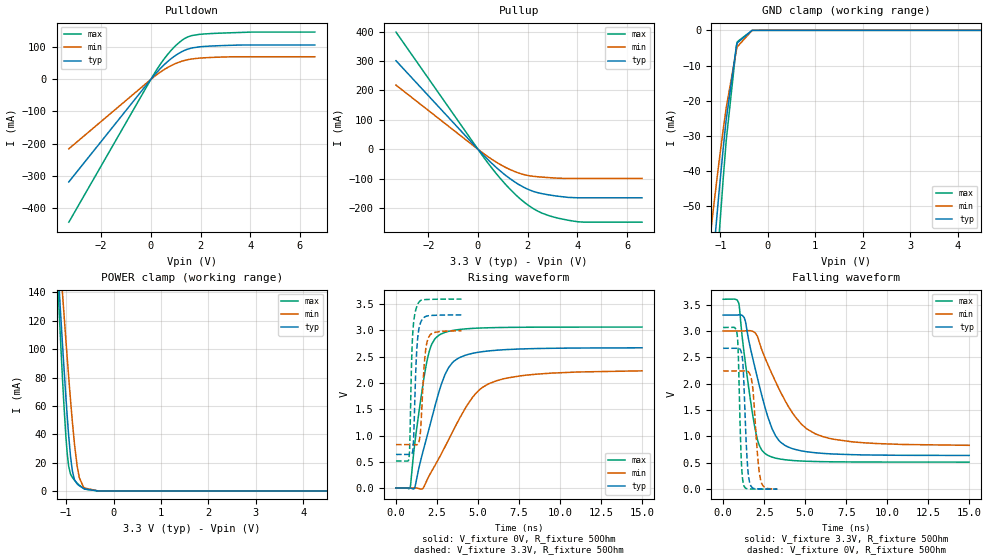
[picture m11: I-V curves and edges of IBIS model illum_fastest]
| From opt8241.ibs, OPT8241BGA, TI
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|   illum_fastest Model
[Model]   illum_fastest
Model_type   I/O
Polarity   Non-Inverting
Enable   Active-High
Vinl  = 0.99
Vinh  = 2.31
Vmeas = 1.65
Vref  = 0
Cref  = 2pF
Rref  = 50
|   typ   min   max
|   (nom PVT)   (fast PVT)   (slow PVT)
C_comp   2.708e-12   2.507e-12   2.914e-12
[Model spec]
|subparameter
Vinl   0.99   0.90   1.08
Vinh   2.31   2.10   2.52
| Where nom  PVT is Nominal Process, 3.3V, 27C
|   Fast PVT is Strong Process,  3.6V, -40C
|   Slow PVT is Weak Process,   3V, 125C
[Voltage Range]   3.3   3   3.6
|Junction Temperature
[Temperature Range]   27   125   -40
[Pullup Reference]   3.3   3   3.6
[Pulldown Reference]   0   0   0
[Power Clamp Reference]   3.3   3   3.6
[GND Clamp Reference]   0   0   0
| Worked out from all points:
|   slope of the pulldown table from 0 to 0.495 V, typ, clamps not added: 11.6 ohm
|   slope of the pullup table from 0 to 0.495 V, typ, clamps not added: 11.6 ohm
|   falling waveform, V_fixture 3.3V, R_fixture 50Ohm: 20-80 % time 1.36ns typ, 2.23ns min, 828ps max; typ from 3.3 V to 0.64 V
|   rising waveform, V_fixture 0V, R_fixture 50Ohm: 20-80 % time 1.44ns typ, 2.41ns min, 853ps max; typ from 0 V to 2.67 V
|   rising waveform, V_fixture 3.3V, R_fixture 50Ohm: 20-80 % time 199ps typ, 252ps min, 166ps max; typ from 0.639 V to 3.3 V
|   falling waveform, V_fixture 0V, R_fixture 50Ohm: 20-80 % time 221ps typ, 314ps min, 165ps max; typ from 2.67 V to 0.001 V
[Pulldown]
|   Voltage   I(typ)   I(min)   I(max)
-3.3V     -319.9mA   -216.5mA   -445.5mA
189mV     17.58mA    11.85mA    24.51mA
462mV     40.27mA    27mA       56.22mA
775.2mV   62.22mA    41.4mA     87.06mA
1.056V    78.05mA    51.51mA    109.5mA
1.251V    86.82mA    56.93mA    122mA
1.596V    97.13mA    63.25mA    135.8mA
2.165V    103mA      67.59mA    142mA
4.032V    107.5mA    70.78mA    147.8mA
6.6V      107.5mA    70.78mA    147.8mA
[GND Clamp]
|   Voltage   I(typ)   I(min)   I(max)
-3.3V     -1.553A    -1.315A    -1.789A
-1.214V   -75.2mA    -58.77mA   -96.04mA
-1.133V   -62.06mA   -49.14mA   -79.22mA
-1.033V   -46.78mA   -37.93mA   -59.46mA
-940.5mV  -33.68mA   -28.26mA   -42.33mA
-876mV    -25.29mA   -22mA      -31.29mA
-663mV    -4.673mA   -5.695mA   -4.527mA
-643.2mV  -3.575mA   -4.674mA   -3.252mA
-330mV    -4.518uA   -17.28uA   -5.664uA
6.6V      0A         0A         0A
[Pullup]
|   Voltage   I(typ)   I(min)   I(max)
-3.3V     301mA      218.2mA    398.3mA
1.2mV     -109.4uA   -79.25uA   -144.7uA
459mV     -39.81mA   -28.44mA   -53.04mA
855mV     -70.54mA   -49.65mA   -94.7mA
1.251V    -97.42mA   -67.29mA   -132mA
1.899V    -131.4mA   -86.9mA    -182.2mA
2.237V    -143.2mA   -91.82mA   -202mA
2.565V    -150.5mA   -94.39mA   -216.4mA
3.032V    -157.2mA   -97.16mA   -229.8mA
3.633V    -163.4mA   -99.07mA   -241mA
4.3V      -164.7mA   -99.07mA   -247.6mA
6.6V      -164.7mA   -99.07mA   -247.6mA
[POWER Clamp]
|   Voltage   I(typ)   I(min)   I(max)
-3.3V     1.469A     1.283A     1.789A
-1.219V   185.1mA    209mA      179.1mA
-1.136V   137.8mA    168.8mA    120.5mA
-1.068V   100mA      136.4mA    75.26mA
-1.007V   68.16mA    108.2mA    40.34mA
-973.5mV  52.09mA    93.27mA    25.99mA
-942mV    38.22mA    79.55mA    17.05mA
-867.9mV  14.43mA    49.44mA    9.533mA
-768mV    5.044mA    18.06mA    5.581mA
-720mV    3.634mA    9.339mA    4.032mA
-606mV    1.373mA    2.011mA    1.268mA
6.6V      0A         0A         0A
[Ramp]
R_load = 50
|   typ   min   max
dV/dt_r   1.60207/1.44199e-09   1.33887/2.41367e-09   1.8391/8.51662e-10
dV/dt_f   1.59624/1.35443e-09   1.30098/2.22249e-09   1.85169/8.27508e-10
[Falling Waveform]
V_fixture = 3.3V
V_fixture_min = 3V
V_fixture_max = 3.6V
R_fixture = 50Ohm
|   Time   V(typ)   V(min)   V(max)
0s        3.3V       3V         3.6V
940ps     3.305V     3V         3.536V
1.292ns   3.247V     2.999V     2.547V
1.92ns    2.329V     2.971V     1.19V
2.22ns    1.944V     2.771V     819.8mV
2.646ns   1.451V     2.42V      656.3mV
3.516ns   887.3mV    1.832V     569.5mV
4.372ns   754.8mV    1.381V     541.1mV
5.612ns   690.8mV    1.05V      524.9mV
15ns      639.5mV    831.6mV    513.7mV
[Rising Waveform]
V_fixture = 0V
V_fixture_min = 0V
V_fixture_max = 0V
R_fixture = 50Ohm
|   Time   V(typ)   V(min)   V(max)
0s        1.479nV    67.62nV    784.6pV
858ps     1.112mV    -3.387uV   7.553mV
1.152ns   15.08mV    628.1uV    864.6mV
1.848ns   932.1mV    121mV      2.354V
2.186ns   1.333V     325.7mV    2.743V
2.642ns   1.854V     580.2mV    2.914V
3.53ns    2.414V     1.119V     3.005V
4.664ns   2.565V     1.725V     3.04V
5.668ns   2.612V     1.988V     3.052V
15ns      2.67V      2.231V     3.065V
[Rising Waveform]
V_fixture = 3.3V
V_fixture_min = 3V
V_fixture_max = 3.6V
R_fixture = 50Ohm
|   Time   V(typ)   V(min)   V(max)
0s        638.9mV    826.8mV    513.7mV
798ps     639.2mV    826.8mV    574.6mV
844ps     639.3mV    826.8mV    876.2mV
940ps     641.8mV    826.9mV    2.274V
1.012ns   691.8mV    827mV      2.894V
1.314ns   2.829V     828.7mV    3.492V
1.47ns    3.124V     991mV      3.564V
1.75ns    3.257V     2.46V      3.588V
1.964ns   3.281V     2.857V     3.592V
3.994ns   3.297V     2.994V     3.599V
[Falling Waveform]
V_fixture = 0V
V_fixture_min = 0V
V_fixture_max = 0V
R_fixture = 50Ohm
|   Time   V(typ)   V(min)   V(max)
0s        2.671V     2.241V     3.065V
854ps     2.672V     2.241V     2.935V
922ps     2.675V     2.241V     2.569V
1.106ns   2.599V     2.241V     555.8mV
1.268ns   1.984V     2.242V     63.34mV
1.452ns   602.6mV    2.241V     9.233mV
1.618ns   122mV      2.19V      5.284mV
1.816ns   21.23mV    1.886V     3.533mV
2.272ns   4.152mV    193.2mV    1.925mV
3.296ns   1.448mV    3.125mV    632.5uV
